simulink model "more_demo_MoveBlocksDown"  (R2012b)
settings: Solver=ode45  StartTime=0.0  StopTime=10.0  RelTol=1e-3
model workspace (MAT data in the model file):
  MyK = 1.23

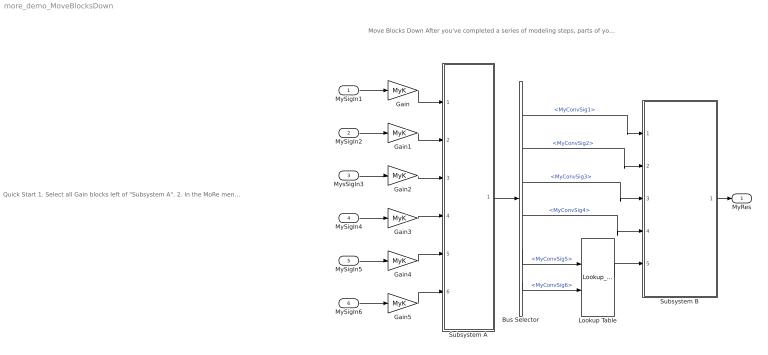
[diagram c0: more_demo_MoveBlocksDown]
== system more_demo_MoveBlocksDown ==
  note: Quick Start 1. Select all Gain blocks left of "Subsystem A". 2. In the MoRe menu select "Partition->Move Blocks Down". 3. In the dialog select "Subsystem A" as the target. 4. Click "Ok" and note the changes. 5. Select the Bus Selector and the Lookup Table between the subsystems. 6. In the MoRe menu select "Partition->Move Blocks Down" again. 7. In the dialog select "Subsystem B" as the target. 8. Click "Ok" and note the changes.
  note: Move Blocks Down After you've completed a series of modeling steps, parts of your model may need to be repartitioned. The "Move Blocks Down" action helps you to move parts of your model into an existing subsystem.
  MySigIn1 : Inport
  MySigIn2 : Inport  Port=2
  MysSigIn3 : Inport  Port=3
  MySigIn4 : Inport  Port=4
  MySigIn5 : Inport  Port=5
  MySigIn6 : Inport  Port=6
  Bus Selector : BusSelector  OutputSignals=MyConvSig1,MyConvSig2,MyConvSig3,MyConvSig4,MyConvSig5,MyConvSig6
  Gain{,1..5} (6 alike) : Gain  Gain=MyK
  Lookup Table : Lookup_n-D  BreakpointsForDimension1=[-5:5]  Table=tanh([-5:5])  RndMeth=Simplest
  Subsystem A : Subsystem
  Subsystem B : Subsystem
  MyRes : Outport
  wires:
  Subsystem B/1(MyRes) -> MyRes/1
  MySigIn6/1 -> Gain5/1
  MySigIn5/1 -> Gain4/1
  MySigIn4/1 -> Gain3/1
  MysSigIn3/1 -> Gain2/1
  MySigIn2/1 -> Gain1/1
  MySigIn1/1 -> Gain/1
  Gain5/1 -> Subsystem A/6(MySig6)
  Gain4/1 -> Subsystem A/5(MySig5)
  Gain3/1 -> Subsystem A/4(MySig4)
  Gain2/1 -> Subsystem A/3(MySig3)
  Gain1/1 -> Subsystem A/2(MySig2)
  Gain/1 -> Subsystem A/1(MySig1)
  Subsystem A/1(MySignals) -> Bus Selector/1
  Lookup Table/1 -> Subsystem B/5(MyLookedUpSig1)
  Bus Selector/6 -> Lookup Table/2  "<MyConvSig6>"
  Bus Selector/5 -> Lookup Table/1  "<MyConvSig5>"
  Bus Selector/4 -> Subsystem B/4(MyConvSig4)  "<MyConvSig4>"
  Bus Selector/3 -> Subsystem B/3(MyConvSig3)  "<MyConvSig3>"
  Bus Selector/2 -> Subsystem B/2(MyConvSig2)  "<MyConvSig2>"
  Bus Selector/1 -> Subsystem B/1(MyConvSig1)  "<MyConvSig1>"

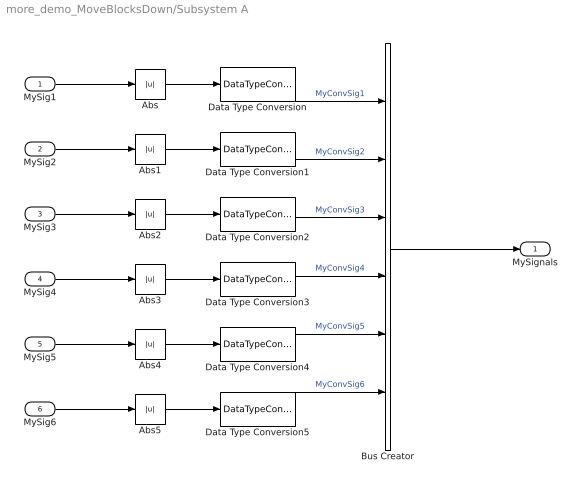
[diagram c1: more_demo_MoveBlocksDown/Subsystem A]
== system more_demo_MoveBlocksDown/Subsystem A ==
  MySig1 : Inport
  MySig2 : Inport  Port=2
  MySig3 : Inport  Port=3
  MySig4 : Inport  Port=4
  MySig5 : Inport  Port=5
  MySig6 : Inport  Port=6
  Abs{,1..5} (6 alike) : Abs
  Bus Creator : BusCreator  Inputs=6
  Data Type Conversion{,1..5} (6 alike) : DataTypeConversion
  MySignals : Outport
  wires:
  Bus Creator/1 -> MySignals/1
  Data Type Conversion/1 -> Bus Creator/1  "MyConvSig1"
  Abs/1 -> Data Type Conversion/1
  Data Type Conversion1/1 -> Bus Creator/2  "MyConvSig2"
  Abs1/1 -> Data Type Conversion1/1
  Data Type Conversion2/1 -> Bus Creator/3  "MyConvSig3"
  Abs2/1 -> Data Type Conversion2/1
  Data Type Conversion3/1 -> Bus Creator/4  "MyConvSig4"
  Abs3/1 -> Data Type Conversion3/1
  Data Type Conversion4/1 -> Bus Creator/5  "MyConvSig5"
  Abs4/1 -> Data Type Conversion4/1
  Data Type Conversion5/1 -> Bus Creator/6  "MyConvSig6"
  Abs5/1 -> Data Type Conversion5/1
  MySig6/1 -> Abs5/1
  MySig5/1 -> Abs4/1
  MySig4/1 -> Abs3/1
  MySig3/1 -> Abs2/1
  MySig2/1 -> Abs1/1
  MySig1/1 -> Abs/1

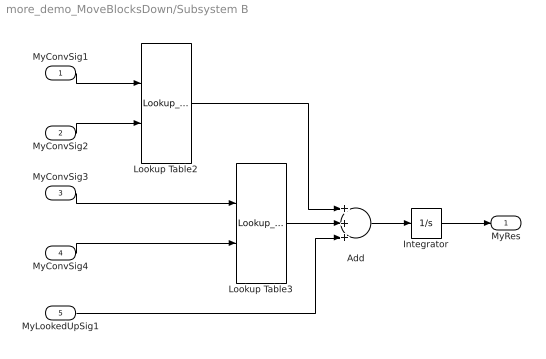
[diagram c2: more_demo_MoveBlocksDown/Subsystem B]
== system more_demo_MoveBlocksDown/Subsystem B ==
  MyConvSig1 : Inport
  MyConvSig2 : Inport  Port=2
  MyConvSig3 : Inport  Port=3
  MyConvSig4 : Inport  Port=4
  MyLookedUpSig1 : Inport  Port=5
  Add : Sum  Inputs=+++
  Integrator : Integrator
  Lookup Table2 : Lookup_n-D  BreakpointsForDimension1=[-5:5]  Table=tanh([-5:5])  RndMeth=Simplest
  Lookup Table3 : Lookup_n-D  BreakpointsForDimension1=[-5:5]  Table=tanh([-5:5])  RndMeth=Simplest
  MyRes : Outport
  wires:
  Lookup Table3/1 -> Add/2
  Integrator/1 -> MyRes/1
  Add/1 -> Integrator/1
  Lookup Table2/1 -> Add/1
  MyLookedUpSig1/1 -> Add/3
  MyConvSig4/1 -> Lookup Table3/2
  MyConvSig3/1 -> Lookup Table3/1
  MyConvSig2/1 -> Lookup Table2/2
  MyConvSig1/1 -> Lookup Table2/1
